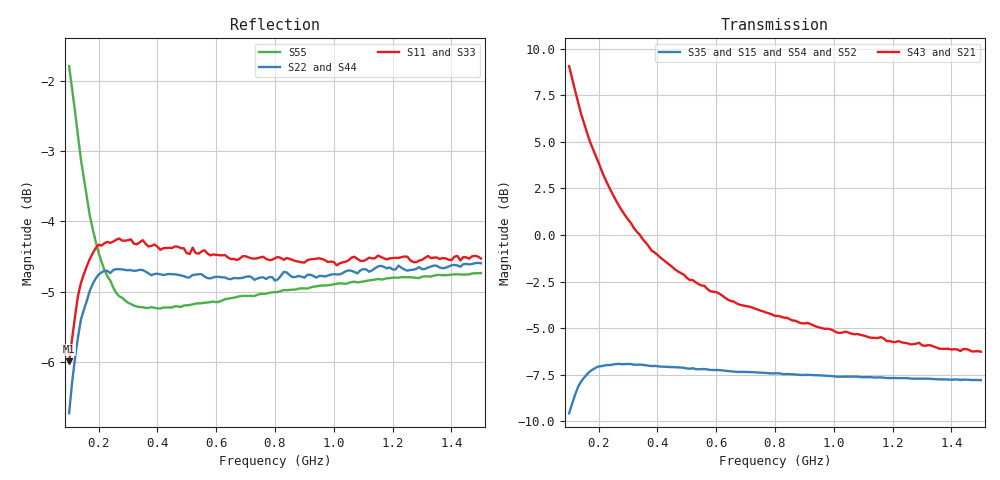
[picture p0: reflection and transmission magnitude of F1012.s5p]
!  POLYFET RF DEVICES
!  S PARAMETERS FOR
!  F1012 (Each Side)
!  VDS=28, IDQ=600mA
! Date: Mon Oct 21 16:54:45 1991
! Bias (V mA) : V1=1.9979000  I1=0.0040389  V2=27.992500  I2=661.20100
!AWR Design Environment (2053) Wed Feb 04 14:27:37 2004
!freq-unit  param-type  data-format  keyword  impedance-ohms
# MHz  S  MA  R  50
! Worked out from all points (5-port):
!   141 points, 100 MHz to 1.5 GHz, reference 50 ohm
!   strongest paths, dB at 100 MHz, 450 MHz, 800 MHz, 1.15 GHz, 1.5 GHz:
!     S43: 9.1, -1.7, -4.3, -5.5, -6.3
!     S21: 9.1, -1.7, -4.3, -5.5, -6.3
!     S35: -9.6, -7.1, -7.4, -7.6, -7.8
!     S15: -9.6, -7.1, -7.4, -7.6, -7.8
!     S54: -9.6, -7.3, -7.6, -7.7, -7.7
!     S52: -9.6, -7.3, -7.6, -7.7, -7.7
!   lowest |S11| = -6.0 dB at 100 MHz (marker M1), VSWR 3.01, Z = 23 - j28.6 ohm
!   |S11| at or under -10 dB: nowhere
